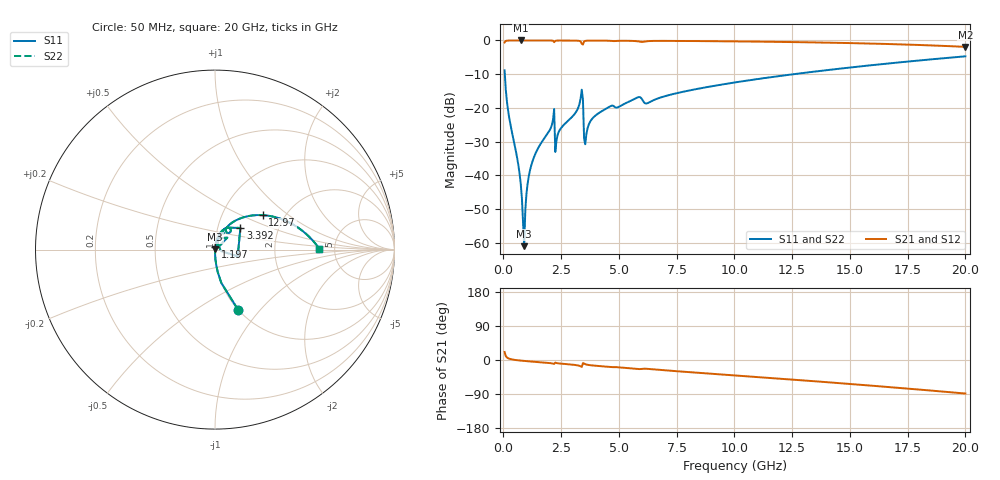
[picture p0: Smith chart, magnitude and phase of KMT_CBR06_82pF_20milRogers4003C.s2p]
! Data measured by Modelithics Inc. support@modelithics.com 813-866-6335
! KEMET CBR0603 82pF, Pad Width= 0.851mm, Pad Length= 0.64mm, Pad Gap= 0.62mm, 20mil Rogers 4003C substrate Data, January 2022
# hz S ma R 50
! 2 Port Network Data from SP1.SP block
! freq  magS11  angS11  magS21  angS21  magS12  angS12  magS22  angS22
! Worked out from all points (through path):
!   401 points, 50 MHz to 20 GHz, reference 50 ohm
!   highest |S21| = -0.01 dB at 748.2 MHz (marker M1); lowest = -1.9 dB at 20 GHz (marker M2)
!   group delay of S21, straight-line fit = 12.4 ps
!   lowest |S11| = -61.1 dB at 897.9 MHz (marker M3), VSWR 1.00, Z = 50.1 + j0.0622 ohm
!   |S11| at or under -10 dB: 59.9 MHz to 12.58 GHz (12.52 GHz wide, 198 % of centre)
!   |S22| runs from -61.1 to -4.7 dB; largest |S21 - S12| = 0
!   S11 on the Smith chart (normalised r, x): 50 MHz: 1.00, -0.77; 1.197 GHz: 1.00, +0.03; 3.392 GHz: 1.28, +0.32; 12.97 GHz: 1.55, +0.67; 20 GHz: 3.78, +0.06
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5e7  0.3598 -69.0  0.9327 21.0  0.9327 21.0  0.3598 -69.0
2.495e8  0.07123 -86.3  0.9971 3.4  0.9971 3.4  0.07123 -86.3
5.98625e8  0.0176 -89.0  0.9993 -0.6  0.9993 -0.6  0.0176 -89.0
7.4825e8  0.007438 -87.4  0.9994 -1.6  0.9994 -1.6  0.007438 -87.4
7.98125e8  0.00459 -84.8  0.9994 -1.9  0.9994 -1.9  0.00459 -84.8
8.97875e8  0.0008844 44.6  0.9994 -2.5  0.9994 -2.5  0.0008844 44.6
9.4775e8  0.003106 75.8  0.9993 -2.7  0.9993 -2.7  0.003106 75.8
1.0475e9  0.007558 81.8  0.9993 -3.3  0.9993 -3.3  0.007558 81.8
1.197125e9  0.01373 83.1  0.9992 -4.0  0.9992 -4.0  0.01373 83.1
2.094875e9  0.05528 78.0  0.9954 -8.8  0.9954 -8.8  0.05528 78.0
2.34425e9  0.0396 77.7  0.9966 -8.6  0.9966 -8.6  0.0396 77.7
3.34175e9  0.1384 62.2  0.9641 -16.8  0.9641 -16.8  0.1384 62.2
3.391625e9  0.1858 40.6  0.891 -18.3  0.891 -18.3  0.1858 40.6
3.591125e9  0.04083 66.4  0.9908 -12.0  0.9908 -12.0  0.04083 66.4
3.8405e9  0.06876 73.5  0.9948 -14.3  0.9948 -14.3  0.06876 73.5
4.588625e9  0.1039 68.4  0.9885 -18.3  0.9885 -18.3  0.1039 68.4
6.73325e9  0.1396 61.9  0.9851 -26.1  0.9851 -26.1  0.1396 61.9
1.0025e10  0.2382 48.8  0.9684 -40.6  0.9684 -40.6  0.2382 48.8
1.296762e10  0.3285 35.7  0.941 -53.7  0.941 -53.7  0.3285 35.7
1.336662e10  0.3415 33.9  0.9362 -55.6  0.9362 -55.6  0.3415 33.9
1.670825e10  0.4567 17.9  0.884 -71.5  0.884 -71.5  0.4567 17.9
2e10  0.5812 0.5  0.8026 -88.5  0.8026 -88.5  0.5812 0.5
